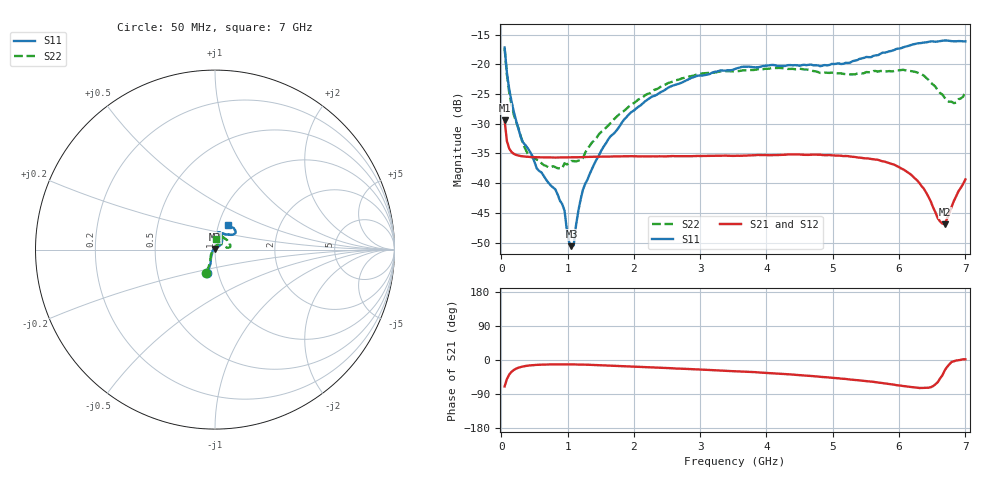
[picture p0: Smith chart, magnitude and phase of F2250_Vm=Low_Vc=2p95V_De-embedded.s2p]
! Integrated Device Technology
! Corporate Headquarters
! 6024 Silver Creek Valley Road
! San Jose, CA 95138  USA
! Phone:  1-408-284-8200
! Toll Free:  1-800-223-1366
! Webpage:  http://www.idt.com/
! Timing and RF Division
! 515 Groton Road, Suite 102
! Westford, MA 01886-6024
! Device:  F2250
! Description: Voltage Variable RF Attenuator
! Frequency:  50.0 -  6000.00 MHz
! Package:  3x3 mm Thin QFN Plastic Package: 16 pin
! Ports:  2 RF, 3 DC
!  Pin  1  = GND
!  Pin  2  = NC
!  Pin  3  = RF1  = Port 1
!  Pin  4  = NC
!  Pin  5  = GND
!  Pin  6  = GND
!  Pin  7  = GND
!  Pin  8  = GND
!  Pin  9  = NC
!  Pin 10  = RF2  = Port 2
!  Pin 11  = NC
!  Pin 12  = GND
!  Pin 13  = GND
!  Pin 14  = VCNTRL
!  Pin 15  = VDD
!  Pin 16  = VMODE
! Vcntrl:  2.950 Volts
! Vmode:  +0.000 Volts
! Vdd:  +3.30  Volts
! Current:  1.176 mA
! Data:  The device was measured on a the F2250 evaluation board which has
!  individual transmission lines to the RF pins.  Data was collected
!  using a calibrated network analyzer.  The evaluation board was
!  de-embedded using a TRL calibration technique.
!  The reference plane is the edge of the package pin.
! Misc:  SN 10
!  Action Tracker AT0258
! Date Measured:  2014-11-26
! Date:  2015-10-15  MJV
! Note:
!  Integrated Device Technology supplies this data as a sample of measured
!  data at the package pin for this product.  Your particular data for this
!  product may vary.
!  Data was taken at 25 degrees C.
!  Integrated Device Technology reserves the right to change this data at anytime.
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# GHz S dB R 50
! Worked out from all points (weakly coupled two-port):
!   201 points, 50 MHz to 7 GHz, reference 50 ohm
!   highest |S21| = -29.41 dB at 50 MHz (marker M1); lowest = -46.9 dB at 6.687 GHz (marker M2)
!   lowest |S11| = -50.6 dB at 1.058 GHz (marker M3), VSWR 1.01, Z = 49.8 + j0.245 ohm
!   |S11| at or under -10 dB: start of sweep to end of sweep
!   |S22| runs from -37.5 to -17.3 dB; largest |S21 - S12| = 6.3e-05
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0.05  -17.18 -108.6  -29.41 -69.8  -29.41 -69.8  -17.28 -111.0
0.08475  -21.45 -107.4  -32.92 -50.4  -32.92 -50.3  -21.75 -110.2
0.15425  -26.23 -116.6  -34.76 -31.2  -34.75 -31.1  -26.81 -122.4
0.29325  -32.22 -127.9  -35.44 -18.5  -35.43 -18.5  -32.09 -137.4
0.3975  -34.10 -141.9  -35.56 -15.0  -35.56 -15.0  -35.03 -160.4
0.91875  -43.51 157.9  -35.69 -11.5  -35.68 -11.5  -37.52 133.5
0.9535  -44.60 170.1  -35.69 -11.5  -35.69 -11.5  -36.64 131.1
1.023  -49.94 143.4  -35.67 -11.6  -35.67 -11.6  -36.64 115.9
1.05775  -50.60 123.7  -35.67 -11.6  -35.67 -11.6  -36.28 110.7
1.0925  -50.45 89.9  -35.66 -11.7  -35.66 -11.7  -36.29 106.5
1.162  -44.66 57.3  -35.64 -11.9  -35.64 -11.9  -36.22 95.6
1.2315  -41.09 44.4  -35.61 -12.1  -35.60 -12.1  -35.81 85.7
1.6485  -32.10 42.0  -35.52 -14.6  -35.51 -14.6  -29.88 64.4
1.96125  -28.04 42.2  -35.46 -17.2  -35.47 -17.2  -26.81 56.8
2.37825  -24.86 47.3  -35.48 -20.3  -35.48 -20.3  -23.98 56.7
3.525  -20.79 72.4  -35.40 -29.5  -35.40 -29.5  -21.19 74.7
4.7065  -20.17 72.3  -35.20 -42.6  -35.19 -42.7  -21.14 72.2
5.85325  -17.81 40.5  -36.63 -63.4  -36.63 -63.5  -21.14 23.1
6.27025  -16.50 40.0  -39.50 -72.8  -39.50 -72.8  -21.37 9.7
6.68725  -15.99 48.7  -46.90 -27.7  -46.89 -27.5  -25.63 28.7
6.861  -16.13 55.1  -42.20 -1.4  -42.16 -1.4  -26.45 57.9
7  -16.14 63.2  -39.37 1.9  -39.33 1.7  -24.63 83.1
